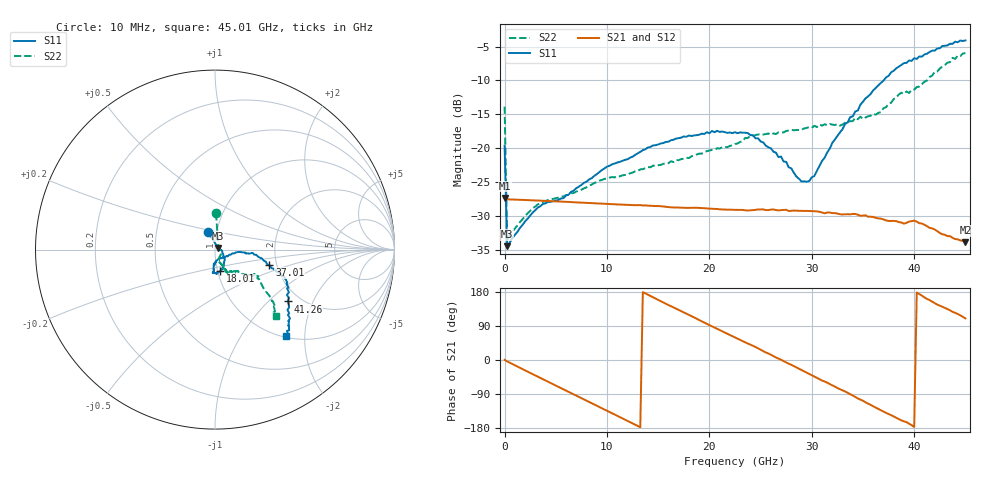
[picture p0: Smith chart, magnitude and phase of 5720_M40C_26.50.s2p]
! Device:  ADRF5720
! Description: 0.5dB LSB GaAs MMIC 6-bit Digital Attenuator
! Frequency:  0.000009 -  40 GHz
! Ports:
!	RF1	= Port 1
!	RF2	= Port 2
! Vdd:  3.3 Volt
! Vss:  -3.3 Volt
! Control:  0/3.3 Volt
! State:  26.50 dB attenuation
! Data:  The device was measured using G-S-G Probes on a matrix board.
!  Data was collected using an calibrated 4 port network analyzer.
!  The reference plane for this measurement is at the launchers.
! Note:  Analog Devices supplies this data as a sample of measured data
!  for this product.  Your particular data for this product may vary.
!  Data was taken at -40 degrees C.
!  Analog Devices reserves the right to change this data at anytime.
# GHZ S DB R 45.0
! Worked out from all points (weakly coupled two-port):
!   181 points, 10 MHz to 45.01 GHz, reference 45 ohm
!   highest |S21| = -27.36 dB at 10 MHz (marker M1); lowest = -33.9 dB at 45.01 GHz (marker M2)
!   lowest |S11| = -34.5 dB at 260 MHz (marker M3), VSWR 1.04, Z = 46.5 + j0.897 ohm
!   |S11| at or under -10 dB: start of sweep to 37.03 GHz
!   |S22| runs from -33.6 to -6.0 dB; largest |S21 - S12| = 0.00023
!   S11 on the Smith chart (normalised r, x): 10 MHz: 0.91, +0.18; 18.01 GHz: 1.03, -0.25; 37.01 GHz: 1.83, -0.35; 41.26 GHz: 1.72, -1.32; 45.01 GHz: 1.02, -1.61
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0.01  -19.63 111.1  -27.36 0.4  -27.38 0.4  -13.87 88.4
0.26  -34.46 30.6  -27.54 -3.7  -27.56 -3.7  -33.56 23.0
3.26  -28.75 -5.7  -27.73 -44.2  -27.75 -44.2  -28.28 -28.6
5.76  -27.37 -19.7  -27.90 -77.4  -27.92 -77.4  -27.13 -47.9
7.76  -25.11 -33.4  -28.05 -104.0  -28.07 -104.0  -25.92 -62.0
10.01  -22.72 -43.3  -28.22 -134.0  -28.24 -134.0  -24.44 -68.1
15.26  -19.31 -65.5  -28.56 155.2  -28.58 155.2  -22.46 -70.4
18.01  -18.13 -76.6  -28.81 119.1  -28.84 119.0  -21.46 -67.3
22.76  -17.79 -94.6  -29.11 56.3  -29.13 56.3  -19.30 -65.2
24.76  -18.54 -93.2  -29.04 30.8  -29.06 30.7  -17.98 -62.1
27.01  -21.23 -91.8  -29.14 0.7  -29.16 0.6  -17.69 -63.5
29.01  -24.91 -73.6  -29.25 -26.3  -29.27 -26.4  -17.26 -62.9
30.26  -24.11 -41.2  -29.31 -43.3  -29.33 -43.5  -16.70 -61.6
33.26  -16.42 -5.4  -29.76 -83.0  -29.78 -83.1  -16.24 -53.2
36.26  -11.11 -12.9  -30.28 -125.7  -30.30 -125.9  -15.05 -43.0
37.01  -10.03 -15.9  -30.51 -136.5  -30.53 -136.6  -14.09 -41.0
37.76  -8.80 -19.6  -30.74 -145.5  -30.76 -145.8  -13.29 -40.0
39.26  -7.41 -22.5  -31.01 -163.9  -31.04 -164.1  -11.63 -32.8
40.01  -6.73 -27.2  -30.69 -176.8  -30.72 -177.0  -11.35 -32.4
41.26  -6.06 -35.5  -31.50 161.2  -31.51 161.1  -10.01 -36.1
43.76  -4.59 -45.7  -33.23 127.0  -33.22 126.8  -6.66 -43.5
45.01  -4.10 -50.7  -33.88 109.8  -33.98 109.8  -5.97 -47.4
